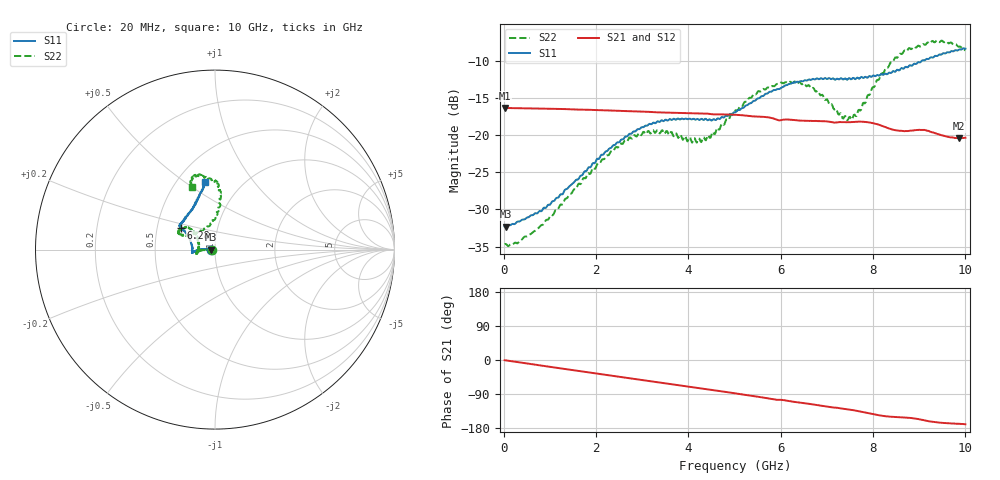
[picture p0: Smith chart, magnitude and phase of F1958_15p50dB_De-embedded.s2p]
! Integrated Device Technology
! Corporate Headquarters
! 6024 Silver Creek Valley Road
! San Jose, CA 95138  USA
! Phone:  1-408-284-8200
! Toll Free:  1-800-223-1366
! Webpage:  http://www.idt.com/
! Timing and RF Division
! 515 Groton Road, Suite 102
! Westford, MA 01886-6024
! Device:  F1958
! Description: 7-bit 0.25 dB Digital Step Attenuator
! Frequency:  0.001 -  6.000 GHz
! Package:  4x4 mm Thin QFN Plastic Package: 24 pin
! Ports:  2 RF, 12 DC
!  Pin  1  = D0
!  Pin  2  = VDD
!  Pin  3  = VMODE
!  Pin  4  = GND
!  Pin  5  = RF1  =  Port 1
!  Pin  6  = GND
!  Pin  7  = GND
!  Pin  8  = GND
!  Pin  9  = GND
!  Pin 10  = GND
!  Pin 11  = GND
!  Pin 12  = GND
!  Pin 13  = GND
!  Pin 14  = RF2  =  Port 2
!  Pin 15  = GND
!  Pin 16  = LE
!  Pin 17  = CLK
!  Pin 18  = DATA
!  Pin 19  = D6
!  Pin 20  = D5
!  Pin 21  = D4
!  Pin 22  = D3
!  Pin 23  = D2
!  Pin 24  = D1
! State:  62
! Atten State:  15.50 dB
! Voltage:  +3.30 Volts
! Current:  0.258 mA
! Data:  The device was measured on a F1958 evaluation board which has
!  individual transmission lines to the RF pins.  Data was collected
!  using a calibrated network analyzer.  The evaluation board was
!  de-embedded using Automatic Fixture Removal (AFR).
!  The reference plane is the edge of the package pin.
! Misc:
!  Action Tracker AT0419
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# GHz S dB R 50
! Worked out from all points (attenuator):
!   500 points, 20 MHz to 10 GHz, reference 50 ohm
!   highest |S21| = -16.36 dB at 20 MHz (marker M1); lowest = -20.4 dB at 9.86 GHz (marker M2)
!   lowest |S11| = -32.3 dB at 40 MHz (marker M3), VSWR 1.05, Z = 47.6 - j0.0735 ohm
!   |S11| at or under -10 dB: start of sweep to 9.059 GHz
!   |S22| runs from -34.9 to -7.3 dB; largest |S21 - S12| = 0.00051
!   S11 on the Smith chart (normalised r, x): 20 MHz: 0.95, -0.00; 6.28 GHz: 0.66, +0.17; 10 GHz: 0.68, +0.60
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0.02  -32.29 -178.1  -16.36 -0.5  -16.35 -0.4  -34.70 -177.6
0.04  -32.32 -178.2  -16.36 -0.8  -16.36 -0.8  -34.64 -176.6
0.32  -31.62 177.3  -16.41 -5.9  -16.40 -5.9  -34.44 178.7
0.72  -30.54 177.2  -16.44 -13.0  -16.44 -13.0  -32.66 -179.9
1.7  -25.40 177.3  -16.59 -30.3  -16.59 -30.2  -26.15 -180.0
2.6  -20.49 -178.5  -16.78 -46.0  -16.76 -46.1  -20.97 -175.2
2.92  -19.21 -175.5  -16.84 -51.6  -16.83 -51.7  -19.78 -171.7
3.36  -18.23 -172.9  -16.96 -59.3  -16.96 -59.5  -19.62 -167.1
4.3  -17.86 -178.3  -17.11 -75.6  -17.13 -75.6  -20.66 164.7
4.64  -17.75 173.2  -17.23 -81.3  -17.24 -81.3  -19.07 151.9
5.02  -16.94 162.0  -17.28 -88.2  -17.30 -88.2  -16.69 140.6
5.54  -15.04 151.6  -17.54 -97.6  -17.55 -97.6  -14.13 141.8
6.28  -12.95 148.0  -17.99 -110.2  -18.00 -110.2  -12.90 152.6
6.68  -12.51 145.9  -18.11 -116.8  -18.13 -116.7  -13.72 155.5
7.32  -12.39 140.3  -18.28 -128.0  -18.28 -127.9  -17.39 135.5
7.5  -12.40 137.2  -18.28 -131.1  -18.28 -131.0  -17.56 117.6
7.7  -12.44 133.2  -18.20 -135.4  -18.20 -135.4  -16.61 100.6
8.34  -11.63 118.3  -19.11 -149.3  -19.11 -149.4  -10.78 83.6
8.68  -10.98 111.6  -19.49 -151.9  -19.48 -151.7  -8.64 87.8
9.26  -9.55 103.7  -19.60 -162.5  -19.60 -162.7  -7.49 100.4
9.86  -8.53 98.9  -20.43 -168.3  -20.47 -168.2  -8.14 109.5
10  -8.40 98.8  -20.37 -169.6  -20.40 -169.5  -8.64 110.3
